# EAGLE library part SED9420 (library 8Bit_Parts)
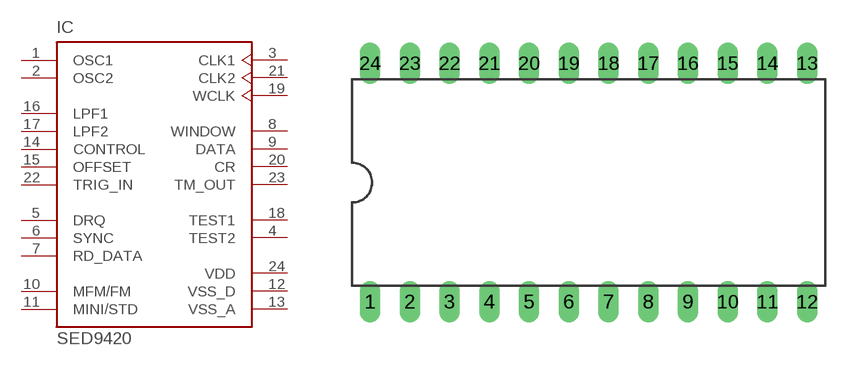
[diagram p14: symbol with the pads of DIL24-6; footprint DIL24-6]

Designator prefix IC

## SED9420  [DIL24-6]
1  OSC1  in
2  OSC2  in
3  CLK1  out
4  TEST2  nc
5  DRQ  in
6  SYNC  in
7  RD_DATA  in
8  WINDOW  out
9  DATA
10  MFM/FM  in
11  MINI/STD  in
12  VSS_D  pwr
13  VSS_A  pwr
14  CONTROL  in
15  OFFSET  in
16  LPF1  in
17  LPF2  in
18  TEST1  nc
19  WCLK  out
20  CR
21  CLK2  out
22  TRIG_IN  in
23  TM_OUT  out
24  VDD  pwr

## Footprint DIL24-6 (pad centres in mm)
Dual In Line Package 0.6 inch
drill 0.813 long: 1 -13.97,-7.62; 2 -11.43,-7.62; 3 -8.89,-7.62; 4 -6.35,-7.62; 5 -3.81,-7.62; 6 -1.27,-7.62; 7 1.27,-7.62; 8 3.81,-7.62; 9 6.35,-7.62; 10 8.89,-7.62; 11 11.43,-7.62; 12 13.97,-7.62; 13 13.97,7.62; 14 11.43,7.62; 15 8.89,7.62; 16 6.35,7.62; 17 3.81,7.62; 18 1.27,7.62; 19 -1.27,7.62; 20 -3.81,7.62; 21 -6.35,7.62; 22 -8.89,7.62; 23 -11.43,7.62; 24 -13.97,7.62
